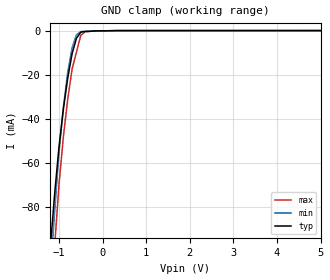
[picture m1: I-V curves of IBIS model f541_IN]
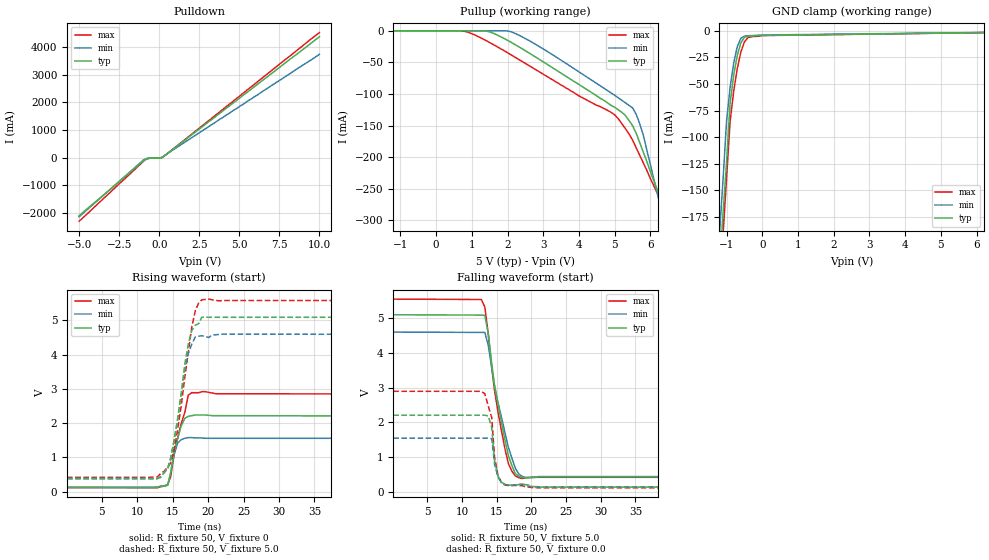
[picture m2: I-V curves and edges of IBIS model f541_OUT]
| TEXAS INSTRUMENTS INCORPORATED
| Standard Linear and Logic Group
| IBIS Model of SN74F541
| OCTAL BUFFERS/DRIVERS WITH 3-STATE OUTPUTS
| SOP 20-pin (NS), SOIC 20-pin (DW), PDIP 20-pin (N) packages.
[IBIS Ver]   3.2
[Comment Char]  |_char
[File Name]   sn74f541.ibs
[File Rev]   2.1 I_die
[Date]   Nov.09, 2004
[Source]   File originated at Texas Instruments, Inc.
[Notes]   The following is a sample IBIS file for the F541.
   - FILE REV HISTORY
   - 2.1 Re-Release IBIS file on 11/09/04
   - Power clamp data deleted as there is no power-clamp diode.
|   - All test data contained in this file are derived from
|   actual measurements.
|   - File created by Nobuhisa Ohtsubo, SLL Product Engineering.
[Disclaimer] Property of Texas Instruments Incorporated.  Unauthorized
   reproduction and/or distribution is strictly prohibited.
   This product is protected under copyright law.
   Created 2000, (C) Copyright 2000, Texas Instruments Inc.,
   All Rights Reserved.
   UNLESS THERE IS A SIGNED, WRITTEN AGREEMENT TO THE
   CONTRARY, TEXAS INSTRUMENTS () IS PROVIDING THE IBIS
   MODELS  AND WITHOUT ANY WARRANTY, EXPRESSED OR
   IMPLIED.  TI assumes no liability for:
   1) the accuracy of the IBIS models provided to your
   company;
   2) the proper functioning of these IBIS Models in your
   design or for any resulting applications; or
   3) infringement of patents, copyrights or intellectual
   property rights resulting from your use of these IBIS
   models.
   TI provides IBIS Models as a service to our customers.
   You and your company shall not distribute, sell or give
   these models to anyone else without prior written
   permission from TI.
   TI reserves the right to make changes to our products or
   to discontinue any semiconductor product or service
   without notice, and advises our customers to obtain the
   latest version of relevant information to verify, before
   placing orders, that the information being relied on is
   current.
   Please be aware that your receipt and use of the IBIS
   information provided shall serve as acceptance of these
   terms and conditions.  If you do not accept these terms,
   you should return or destroy the IBIS models and any
   other accompanying information immediately.
|   Component F541_NS
[Component]   f541_NS
[Manufacturer]  Texas Instruments, Inc.
[Package]
|   typ   min   max
R_pkg   0.044   0.029   0.058
L_pkg   3.666nH   2.317nH   5.115nH
C_pkg   0.548pF   0.316pF   0.725pF
[Pin]   signal_name   model_name   R_pin   L_pin   C_pin
1   1OE_NOT   f541_IN   0.058   5.115nH   0.725pF
2   A1   f541_IN   0.053   4.591nH   0.724pF
3   A2   f541_IN   0.049   3.754nH   0.572pF
4   A3   f541_IN   0.029   2.549nH   0.388pF
5   A4   f541_IN   0.031   2.317nH   0.316pF
6   A5   f541_IN   0.031   2.317nH   0.316pF
7   A6   f541_IN   0.029   2.556nH   0.399pF
8   A7   f541_IN   0.049   3.754nH   0.579pF
9   A8   f541_IN   0.053   4.591nH   0.724pF
10   GND   GND   0.058   5.115nH   0.725pF
11   Y8   f541_OUT   0.058   5.115nH   0.725pF
12   Y7   f541_OUT   0.053   4.591nH   0.724pF
13   Y6   f541_OUT   0.049   3.754nH   0.579pF
14   Y5   f541_OUT   0.029   2.557nH   0.399pF
15   Y4   f541_OUT   0.031   2.317nH   0.316pF
16   Y3   f541_OUT   0.031   2.317nH   0.316pF
17   Y2   f541_OUT   0.029   2.557nH   0.399pF
18   Y1   f541_OUT   0.049   3.754nH   0.579pF
19   2OE_NOT   f541_OUT   0.053   4.591nH   0.724pF
20   VCC   POWER   0.058   5.115nH   0.725pF
|   Component F541_DW
[Component]   f541_DW
[Manufacturer]   Texas Instruments, Inc.
[Package]
|   typ   min   max
R_pkg   3.800e-02   3.300e-02   4.500e-02
L_pkg   5.012e-09   4.110e-09   6.349e-09
C_pkg   7.170e-13   5.300e-13   8.680e-13
[Pin]   signal_name   model_name   R_pin   L_pin   C_pin
1   1OE_NOT   f541_IN   4.200e-02   6.336e-09   8.650e-13
2   A1   f541_IN   4.300e-02   5.542e-09   8.670e-13
3   A2   f541_IN   3.400e-02   4.714e-09   7.320e-13
4   A3   f541_IN   3.400e-02   4.377e-09   5.910e-13
5   A4   f541_IN   3.600e-02   4.130e-09   5.330e-13
6   A5   f541_IN   3.500e-02   4.111e-09   5.300e-13
7   A6   f541_IN   3.400e-02   4.284e-09   5.830e-13
8   A7   f541_IN   3.400e-02   4.634e-09   7.260e-13
9   A8   f541_IN   4.000e-02   5.518e-09   8.650e-13
10   GND   GND   4.300e-02   6.349e-09   8.660e-13
11   Y8   f541_OUT   4.100e-02   6.281e-09   8.610e-13
12   Y7   f541_OUT   4.500e-02   5.561e-09   8.680e-13
13   Y6   f541_OUT   3.300e-02   4.778e-09   7.420e-13
14   Y5   f541_OUT   3.500e-02   4.414e-09   5.960e-13
15   Y4   f541_OUT   3.500e-02   4.110e-09   5.330e-13
16   Y3   f541_OUT   3.600e-02   4.130e-09   5.330e-13
17   Y2   f541_OUT   3.400e-02   4.377e-09   5.910e-13
18   Y1   f541_OUT   3.400e-02   4.714e-09   7.310e-13
19   2OE_NOT   f541_OUT   4.300e-02   5.569e-09   8.680e-13
20   VCC   POWER   4.200e-02   6.308e-09   8.640e-13
|   Component F541_N
[Component]   f541_N
[Manufacturer]   Texas Instruments, Inc.
[Package]
|   typ   min   max
R_pkg   4.300e-02   3.800e-02   5.000e-02
L_pkg   7.384e-09   4.680e-09   1.032e-08
C_pkg   5.100e-13   2.310e-13   8.210e-13
[Pin]   signal_name   model_name   R_pin   L_pin   C_pin
1   1OE_NOT   f541_IN   4.200e-02   9.427e-09   8.100e-13
2   A1   f541_IN   4.600e-02   8.544e-09   4.560e-13
3   A2   f541_IN   4.800e-02   7.163e-09   4.350e-13
4   A3   f541_IN   4.000e-02   4.825e-09   2.610e-13
5   A4   f541_IN   4.000e-02   5.284e-09   6.480e-13
6   A5   f541_IN   4.000e-02   4.686e-09   2.320e-13
7   A6   f541_IN   4.000e-02   6.359e-09   4.890e-13
8   A7   f541_IN   3.800e-02   7.982e-09   4.750e-13
9   A8   f541_IN   4.300e-02   9.403e-09   4.750e-13
10   GND   GND   5.000e-02   1.032e-08   8.050e-13
11   Y8   f541_OUT   5.000e-02   1.028e-08   8.100e-13
12   Y7   f541_OUT   4.300e-02   9.383e-09   4.770e-13
13   Y6   f541_OUT   3.800e-02   7.978e-09   4.760e-13
14   Y5   f541_OUT   4.000e-02   6.302e-09   4.920e-13
15   Y4   f541_OUT   4.000e-02   4.680e-09   2.310e-13
16   Y3   f541_OUT   4.000e-02   5.284e-09   6.480e-13
17   Y2   f541_OUT   4.000e-02   4.822e-09   2.610e-13
18   Y1   f541_OUT   4.700e-02   7.118e-09   4.390e-13
19   2OE_NOT   f541_OUT   4.600e-02   8.492e-09   4.610e-13
20   VCC   POWER   4.300e-02   9.348e-09   8.210e-13
| Models and submodels in the file (2): f541_IN (Input), f541_OUT (3-state)
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|   Model F541_IN
[Model]   f541_IN
Model_type  Input
Polarity   Inverting
Vinl = 0.8
Vinh = 2.0
| variable   typ   min   max
C_comp   1.33pf   1.00pf   1.66pf
[Temperature Range]   25   0   70
[Voltage Range]   5.0   4.75   5.25
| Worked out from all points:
|   GND clamp passes 1 mA (typ) near -0.51 V on its own axis
[GND Clamp]
|   Voltage   I(typ)   I(min)   I(max)
-5V       -1.09A     -1.45A     -1.18A
-1.2V     -98.7mA    -110mA     -123mA
-1.1V     -74.2mA    -82.4mA    -98mA
-1V       -52.8mA    -55.3mA    -69.8mA
-900mV    -35.7mA    -34.9mA    -48.3mA
-800mV    -21.6mA    -18.9mA    -31.2mA
-700mV    -10.5mA    -7.81mA    -17.5mA
-600mV    -3.51mA    -1.95mA    -9.77mA
-500mV    -712uA     -440uA     -2.16mA
-400mV    -387uA     -353uA     -532uA
-100mV    -112uA     -108uA     -114uA
5V        45.3nA     1.88nA     55.6nA
|   Model F541_OUT
[Model]   f541_OUT
Model_type  3-state
Polarity   Non-Inverting
Enable   Active-Low
Vmeas = 1.5v
Cref = 0pf
| variable   typ   min   max
C_comp   5.8pf   4.35pf   7.25pf
[Temperature Range]   25   0   70
[Voltage Range]   5.0   4.5   5.5
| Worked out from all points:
|   slope of the pulldown table from 0 to 0.75 V, typ, clamps not added: 2.84 ohm
|   rising waveform, R_fixture 50, V_fixture 0: 20-80 % time 1.32ns typ, 929ps min, 1.81ns max; typ from 0.121 V to 2.21 V
|   falling waveform, R_fixture 50, V_fixture 5.0: 20-80 % time 2.32ns typ, 2.58ns min, 2.2ns max; typ from 5.1 V to 0.432 V
|   rising waveform, R_fixture 50, V_fixture 5.0: 20-80 % time 2.03ns typ, 1.95ns min, 2.13ns max; typ from 0.388 V to 5.09 V
|   falling waveform, R_fixture 50, V_fixture 0.0: 20-80 % time 771ps typ, 751ps min, 1.02ns max; typ from 2.2 V to 0.127 V
[Pulldown]
|   Voltage   I(typ)   I(min)   I(max)
-5V       -2.1A      -2.14A     -2.3A
-1V       -124mA     -85mA      -139mA
-900mV    -67.6mA    -53.1mA    -85.1mA
-600mV    -11.3mA    -7.04mA    -20mA
200mV     17.1mA     11.5mA     22.1mA
500mV     149mA      147mA      144mA
10V       4.38A      3.74A      4.53A
[Pullup]
|   Voltage   II(typ)   I(min)   I(max)
-5V       98.9nA     1.4nA      202nA
700mV     54.6nA     1.31nA     -109uA
1.4V      -352uA     1.22nA     -15.5mA
2.1V      -18.2mA    -1.56mA    -38.1mA
4.9V      -118mA     -98.4mA    -129mA
5.3V      -134mA     -114mA     -155mA
5.5V      -150mA     -122mA     -173mA
5.8V      -192mA     -165mA     -209mA
6.4V      -283mA     -306mA     -282mA
6.5V      -299mA     -329mA     -295mA
6.6V      -314mA     -353mA     -307mA
10V       -831mA     -1.15A     -722mA
[GND Clamp]
|   Voltage   I(typ)   I(min)   I(max)
-5V       -2.1A      -2.14A     -2.3A
-1.2V     -222mA     -192mA     -247mA
-1.1V     -173mA     -141mA     -193mA
-1V       -124mA     -85mA      -139mA
-900mV    -67.6mA    -53.1mA    -85.1mA
-800mV    -41.7mA    -30.2mA    -56.8mA
-700mV    -23.1mA    -14.9mA    -35.5mA
-600mV    -11.3mA    -7.04mA    -20mA
-500mV    -6.09mA    -4.84mA    -10.4mA
-400mV    -5.09mA    -4.57mA    -6.3mA
0V        -4.28mA    -3.91mA    -4.4mA
10V       4.28uA     391nA      44uA
[Ramp]
| variable   typ   min   max
dV/dt_r   1.230/1.267n   1.014/1.219n   1.428/1.413n
dV/dt_f   2.838/2.401n   2.532/2.618n   3.000/2.237n
R_load = 50
[Rising Waveform]
R_fixture = 50
V_fixture = 0
|   Time   V(typ)   V(min)   V(max)
97.7ps    121mV      130mV      128mV
12.8ns    133mV      136mV      114mV
14.3ns    186mV      201mV      207mV
14.7ns    540mV      537mV      430mV
15.2ns    1.17V      1.08V      1.08V
15.7ns    1.56V      1.42V      1.56V
16.7ns    2.14V      1.56V      2.31V
17.2ns    2.2V       1.58V      2.82V
17.7ns    2.22V      1.58V      2.89V
49.8ns    2.21V      1.56V      2.85V
[Falling Waveform]
R_fixture = 50
V_fixture = 5.0
V_fixture_min = 4.5
V_fixture_max = 5.5
|   Time   V(typ)   V(min)   V(max)
97.7ps    5.1V       4.6V       5.55V
12.8ns    5.09V      4.59V      5.54V
13.3ns    5.08V      4.59V      5.32V
13.8ns    4.55V      4.21V      4.53V
14.7ns    3.06V      3.04V      2.91V
16.2ns    1.5V       1.7V       1.23V
16.7ns    1.03V      1.27V      802mV
17.2ns    748mV      960mV      584mV
18.2ns    439mV      504mV      396mV
49.8ns    432mV      423mV      410mV
[Rising Waveform]
R_fixture = 50
V_fixture = 5.0
V_fixture_min = 4.5
V_fixture_max = 5.5
|   Time   V(typ)   V(min)   V(max)
97.7ps    388mV      380mV      420mV
12.8ns    383mV      381mV      431mV
14.3ns    690mV      676mV      719mV
15.2ns    1.5V       1.49V      1.23V
16.7ns    3.71V      3.57V      3.32V
17.2ns    4.3V       4.03V      4.07V
17.7ns    4.71V      4.31V      4.81V
18.2ns    4.86V      4.52V      5.29V
19.1ns    5.09V      4.55V      5.6V
49.8ns    5.09V      4.59V      5.58V
[Falling Waveform]
R_fixture = 50
V_fixture = 0.0
|   Time   V(typ)   V(min)   V(max)
97.7ps    2.2V       1.54V      2.89V
13.3ns    2.2V       1.54V      2.82V
13.8ns    2.18V      1.54V      2.46V
14.3ns    1.84V      1.52V      2.13V
14.7ns    890mV      789mV      993mV
15.2ns    448mV      411mV      469mV
15.7ns    265mV      255mV      248mV
16.2ns    215mV      201mV      183mV
21.1ns    127mV      134mV      105mV
49.8ns    127mV      135mV      105mV
